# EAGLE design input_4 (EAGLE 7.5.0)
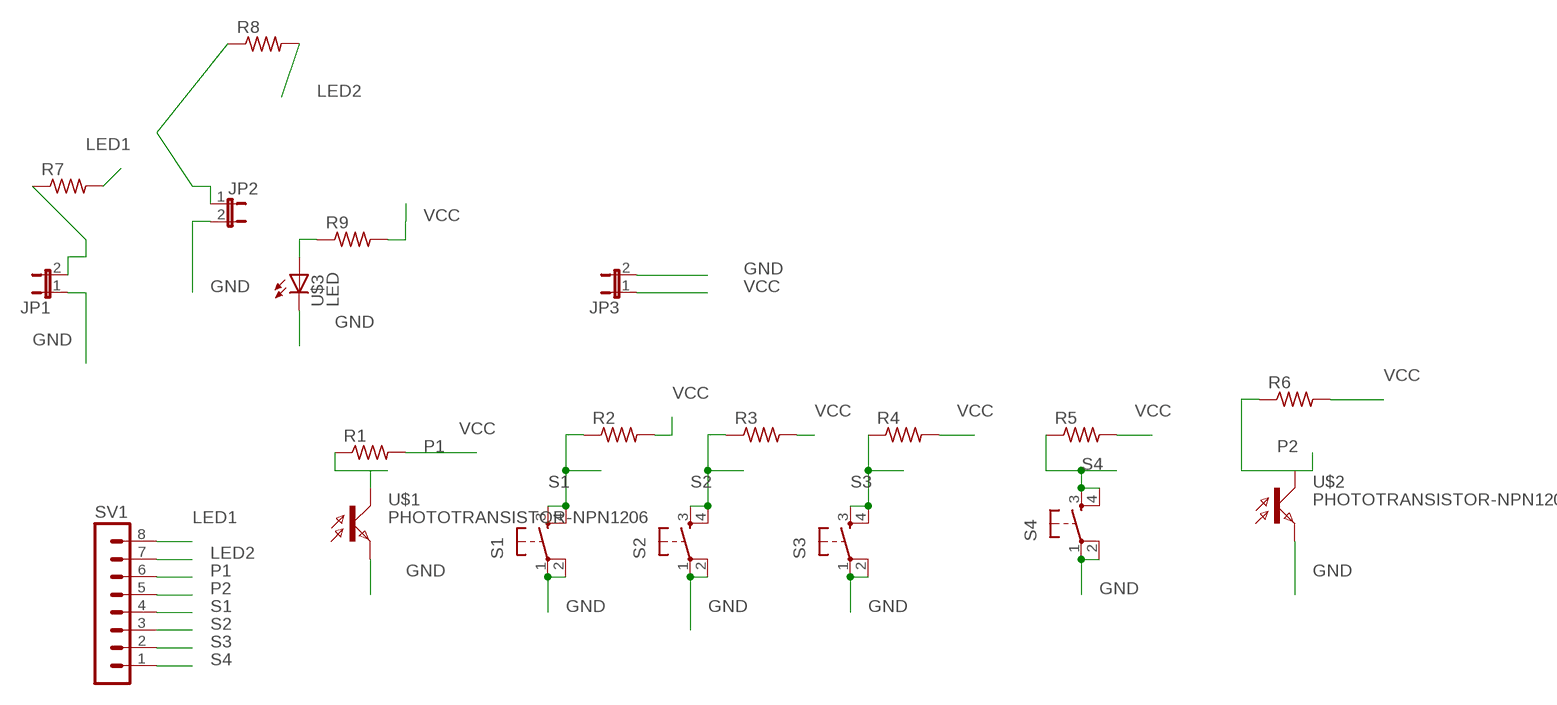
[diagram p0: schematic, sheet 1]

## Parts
JP1  JP1E  [JP1]
JP2  JP1E  [JP1]
JP3  JP1E  [JP1]
R1  RES-US1206FAB  [R1206FAB]
R2  RES-US1206FAB  [R1206FAB]
R3  RES-US1206FAB  [R1206FAB]
R4  RES-US1206FAB  [R1206FAB]
R5  RES-US1206FAB  [R1206FAB]
R6  RES-US1206FAB  [R1206FAB]
R7  RES-US1206FAB  [R1206FAB]
R8  RES-US1206FAB  [R1206FAB]
R9  RES-US1206FAB  [R1206FAB]
S1  6MM_SWITCH6MM_SWITCH  [6MM_SWITCH]
S2  6MM_SWITCH6MM_SWITCH  [6MM_SWITCH]
S3  6MM_SWITCH6MM_SWITCH  [6MM_SWITCH]
S4  6MM_SWITCH6MM_SWITCH  [6MM_SWITCH]
SV1  MA08-1  [MA08-1]
U$1  PHOTOTRANSISTOR-NPN1206  [OP1206]
U$2  PHOTOTRANSISTOR-NPN1206  [OP1206]
U$3  LED  [LED1206]

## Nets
GND: JP1.1 JP2.2 JP3.2 S1.1(P) S1.2(P1) S2.1(P) S2.2(P1) S3.1(P) S3.2(P1) S4.1(P) S4.2(P1) U$1.EMITTER(E) U$2.EMITTER(E) U$3.2(C)
LED1: R7.2 SV1.8
LED2: R8.2 SV1.7
N$15: JP1.2 JP2.1 R7.1 R8.1
N$17: R9.1 U$3.1(A)
P1: R1.1 SV1.6 U$1.COLLECTOR(C)
P2: R6.1 SV1.5 U$2.COLLECTOR(C)
S1: R2.1 S1.3(S) S1.4(S1) SV1.4
S2: R3.1 S2.3(S) S2.4(S1) SV1.3
S3: R4.1 S3.3(S) S3.4(S1) SV1.2
S4: R5.1 S4.3(S) S4.4(S1) SV1.1
VCC: JP3.1 R1.2 R2.2 R3.2 R4.2 R5.2 R6.2 R9.2

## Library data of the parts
JP1-JP3 = jumper:JP1E: JUMPER
R1-R9 = fab:RES-US: Resistor (US Symbol)
S1-S4 = fab:6MM_SWITCH: OMRON SWITCH
SV1 = con-lstb:MA08-1: PIN HEADER; OC_FARNELL: unknown; OC_NEWARK: unknown
U$1 U$2 = fab:PHOTOTRANSISTOR-NPN
U$3 = fab:LED: LED

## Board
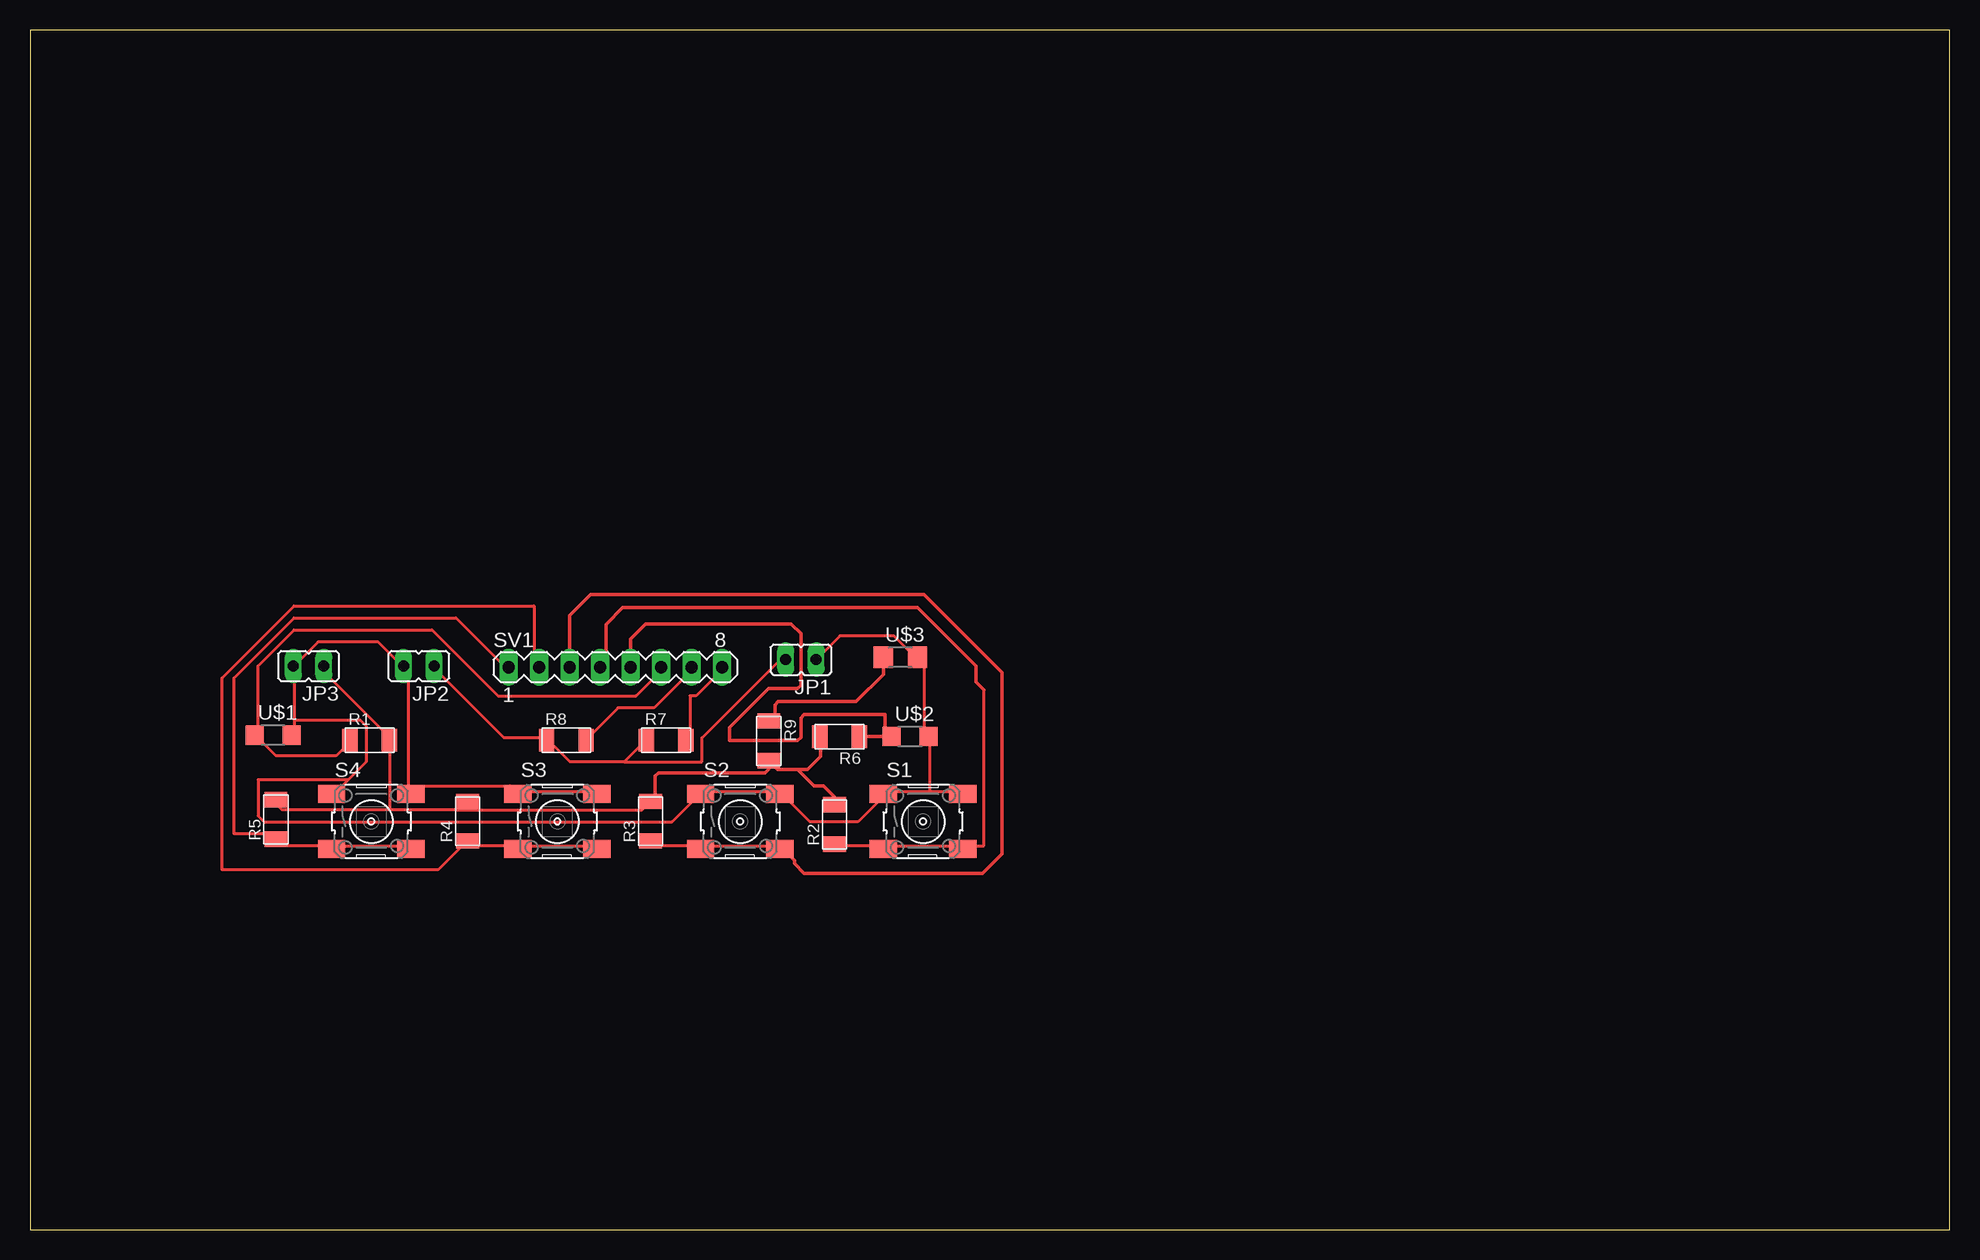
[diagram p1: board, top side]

Size 160 x 100 mm. Coordinates in mm from the lower left corner, seen from the top.
Outline: 0,0 160,0 160,100 0,100 0,0
Copper layers (1*16): Top 0.035mm / dielectric 1.5mm / Bottom 0.035mm
Design rules "default *": minimum track width 10mil, minimum drill 24mil, track to track 16mil, track to pad 16mil, pad to pad 16mil, via to via 16mil, smd to smd 16mil, copper to edge 40mil, drill to drill 8mil, minimum pad ring 10mil, minimum via ring 8mil, stop-mask expansion 4mil, vias tented up to drill 0mil, thermal gap 10mil

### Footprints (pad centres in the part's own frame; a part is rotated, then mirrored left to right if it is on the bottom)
JP1 = drill 0.914 long: 1 0,-1.27; 2 0,1.27
R1206FAB = smd 1.27 x 1.905: 1 -1.651,0; 2 1.651,0
6MM_SWITCH = smd 2.286 x 1.524: 1 -3.302,2.286; 2 3.302,2.286; 3 -3.302,-2.286; 4 3.302,-2.286
MA08-1 = drill 1.016 long: 1 -8.89,0; 2 -6.35,0; 3 -3.81,0; 4 -1.27,0; 5 1.27,0; 6 3.81,0; 7 6.35,0; 8 8.89,0
OP1206 = smd 1.5 x 1.6: COLLECTOR -1.55,0; EMITTER 1.55,0
LED1206 = smd 1.6 x 1.803: 1 -1.422,0; 2 1.422,0

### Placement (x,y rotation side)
JP1  64.26,47.52 90 top
JP2  32.4,46.98 90 top
JP3  23.22,46.98 90 top
R1  28.31,40.79 0 top
R2  67.06,33.77 90 top
R3  51.73,34.04 90 top
R4  36.48,34.04 90 top
R5  20.5,34.19 90 top
R6  67.48,41.08 180 top
R7  53.02,40.79 0 top
R8  44.71,40.79 0 top
R9  61.58,40.74 270 top
S1  74.44,34.02 0 top
S2  59.2,34.02 0 top
S3  43.96,34.02 0 top
S4  28.45,34.02 0 top
SV1  48.79,46.88 0 top
U$1  20.26,41.21 0 top
U$2  73.36,41.1 0 top
U$3  72.55,47.7 0 top

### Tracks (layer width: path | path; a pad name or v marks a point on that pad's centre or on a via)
GND
  Top 0.254: JP1.1 66,48 67.5,49.5 72,49.5 73.5,48 U$3.2 74,47.5 74.5,47.5 74.5,41.5 U$2.EMITTER 75,41 75,36.5 | 75,36.5 77.5,36.5 S1.2 | 75,36.5 71.5,36.5 S1.1 71,36 69,34 65,34 63,36 S2.2 62.5,36.5 56,36.5 S2.1 55.5,36 53.5,34 19.5,34 19,34.5 19,37.5 26.5,37.5 | 22,42.5 22,46.5 JP3.2 22,47 24,49 29,49 31,47 JP2.2 31.5,46.5 31.5,37 | 22,42.5 22,41.5 U$1.EMITTER | 26.5,37.5 28,39 28,42 27.5,42.5 22,42.5 | 26.5,37.5 25.5,36.5 S4.1 | S3.2 47,36.5 41,36.5 S3.1 40.5,36.5 40,37 31.5,37 | 31.5,37 31.5,36.5 S4.2 31.5,37
LED1
  Top 0.254: R7.2 55,41 55,44.5 55.5,44.5 57.5,46.5 SV1.8
LED2
  Top 0.254: R8.2 46.5,41 49,43.5 52,43.5 55,46.5 SV1.7
N$15
  Top 0.254: 49.5,39 45,39 43.5,40.5 R8.1 43,41 39.5,41 34,46.5 JP2.1 | 49.5,39 51,40.5 R7.1 | 49.5,39 56,39 56,41 62.5,47.5 JP1.2
N$17
  Top 0.305: U$3.1 71.13,46.29 68.85,44.01 62.37,44.01 62.1,43.74 62.1,42.91 R9.1
P1
  Top 0.254: R1.1 26.5,40.5 25.5,39.5 20.5,39.5 19,41 U$1.COLLECTOR 19,41.5 19,47 22,50 33.5,50 39,44.5 50.5,44.5 52.5,46.5 SV1.6
P2
  Top 0.305: R6.1 69.15,41.1 U$2.COLLECTOR 71.28,41.63 71.28,42.93 64.53,42.93 64.26,42.66 64.26,41.04 63.99,40.77 58.32,40.77 58.32,41.85 61.56,45.09 63.99,45.09 64.26,45.36 64.26,49.68 63.45,50.49 51.3,50.49 50.06,49.25 SV1.5
S1
  Top 0.254: R2.1 67.5,32 71,32 S1.3 71.5,32 77.5,32 S1.4 78,32 79.5,32 79.5,45 | 48,47 SV1.4
  Top 0.305: 48,47 48,50.43 49.41,51.84 73.98,51.84 78.84,46.98 78.84,45.66 79.5,45
S2
  Top 0.254: R3.1 52,32 55.5,32 S2.3 56,32 62.5,32 S2.4
  Top 0.305: SV1.3 44.98,51.19 46.71,52.92 74.52,52.92 81,46.44 81,31.32 79.38,29.7 64.53,29.7 63.72,30.51 63.72,30.78 63.18,31.32 62.92,31.32 S2.4
S3
  Top 0.254: S3.4 47,32 41,32 S3.3 40.5,32 36.5,32 R4.1 36,32 34,30 16,30 16,46 22,52 42,52 42,47 SV1.2
S4
  Top 0.254: S4.4 31.5,32 25.5,32 S4.3 25,32 21,32 20.5,32.5 R5.1 20.5,33 17,33 17,46 22,51 35.5,51 39.5,47 SV1.1
VCC
  Top 0.254: 35.5,35 30,35 | 30,35 21,35 20.5,35.5 R5.2 | 35.5,35 36,35.5 R4.2 | 30,35 30,40.5 R1.2 30,41 24.5,46.5 JP3.1 | 35.5,35 51,35 51.5,35.5 R3.2
  Top 0.305: R3.2 52.11,35.69 52.11,37.8 52.38,38.07 61.29,38.07 61.56,38.34 61.56,39.07 R9.2 62.33,38.34 63.99,38.34 | R2.2 67.06,36.08 66.15,36.99 65.34,36.99 63.99,38.34 | 63.99,38.34 64.8,38.34 65.88,39.42 65.88,41.03 R6.2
